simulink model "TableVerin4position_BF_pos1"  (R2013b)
settings: Solver=ode15s  StartTime=0.0  StopTime=10  RelTol=1e-3
undefined symbols (not defined in the file): deg, kg, m, mm, N, rad, s, X, Y, Z
libraries: sm_lib x907, fl_lib x24, nesl_utility x18, elec_lib x3, sdl_lib x2, simulink x1
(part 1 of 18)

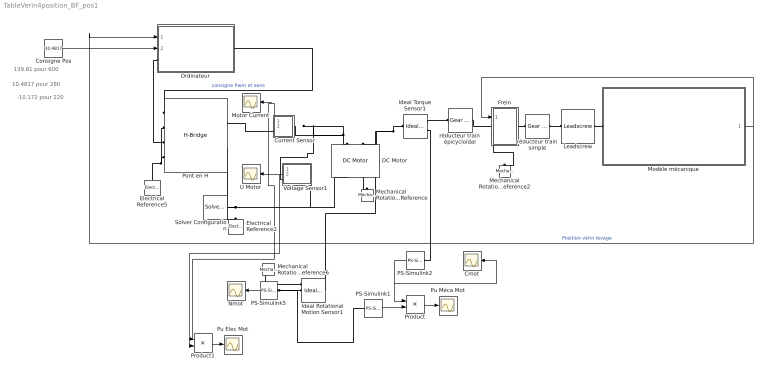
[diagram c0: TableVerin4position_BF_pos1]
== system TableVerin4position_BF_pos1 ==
  note: -10.172 pour 220
  note: 10.4817 pour 280
  note: 139.81 pour 600
  Cmot : Scope
  Consigne Pos : Constant  Value=10.4817
  Current Sensor : Subsystem
  DC Motor : elec_lib/Actuators & Drivers/Rotational Actuators/DC Motor  parameterization=1  Ra=0.53333333 Ohm  La=1600e-6 H  emf_or_torque=2  Kv=0.0637 V/rpm  Ki=0.05555555 N*m/A  T_stall=3e-3*4000/(2*pi*6.25) N*m  w_max=3250 rpm  w_rated=2375 rpm  P_rated=19 W  V_rated=24 V  J=32e-5 kg*m^2  lam_param=2  lam=1e-08 N*m/(rad/s)  i_noload=1.1 A  V_i_noload=24 V  speed0=0 rpm  current_Log=off  voltage_Log=off  power_Log=off  i2r_Log=off  torque_Log=off  speed_Log=off  LocalVarNames=|current|voltage|power|i2r|torque|speed  LocalVarDescs=|Current (A)|Voltage (V)|Power (W)|Electrical losses (W)|Torque (Nm)|Angular speed (rad/s)  LocalVarLogging=[0 0 0 0 0 0]  alpha=0.00393 1/K  Tmeas=25 C  thermal_mass=100 J/K  initial_temperature=25 C
  Electrical Reference2 : fl_lib/Electrical/Electrical Elements/Electrical Reference  i_Log=off  LocalVarNames=|i  LocalVarDescs=|i  LocalVarLogging=[]
  Electrical Reference5 : fl_lib/Electrical/Electrical Elements/Electrical Reference  i_Log=off  LocalVarNames=|i  LocalVarDescs=|i  LocalVarLogging=[]
  Frein : Subsystem
  Ideal Rotational Motion Sensor1 : fl_lib/Mechanical/Mechanical Sensors/Ideal Rotational Motion Sensor  offset=0 deg  w_Log=off  t_Log=off  phi_Log=off  LocalVarNames=|w|t|phi  LocalVarDescs=|w|t|phi  LocalVarLogging=[]
  Ideal Torque Sensor1 : fl_lib/Mechanical/Mechanical Sensors/Ideal Torque Sensor  w_Log=off  t_Log=off  LocalVarNames=|w|t  LocalVarDescs=|w|t  LocalVarLogging=[0 0]
  Leadscrew : sdl_lib/Gears/Rotational- Translational/Leadscrew  Lead=0.008 m  helix_type=1  friction_model=2  friction_parameterization=1  lambda=13 deg  alpha=14.5 deg  fr_coeff=0.08  eff_sn=0.75  eff_ns=0.45  mu_visc=0 N*m/(rad/s)  v_thr=0.001 m/s  LocalVarLogging=[]
  Mechanical Rotational Reference : fl_lib/Mechanical/Rotational Elements/Mechanical Rotational Reference  t_Log=off  LocalVarNames=|t  LocalVarDescs=|t  LocalVarLogging=[]
  Mechanical Rotational Reference2 : fl_lib/Mechanical/Rotational Elements/Mechanical Rotational Reference  t_Log=off  LocalVarNames=|t  LocalVarDescs=|t  LocalVarLogging=[]
  Mechanical Rotational Reference6 : fl_lib/Mechanical/Rotational Elements/Mechanical Rotational Reference  t_Log=off  LocalVarNames=|t  LocalVarDescs=|t  LocalVarLogging=[]
  Modèle mécanique : Subsystem
  Motor Current : Scope
  Nmot : Scope
  Ordinateur : Subsystem
  PS-Simulink1 : nesl_utility/PS-Simulink Converter  PhysicalDomain=network_engine_domain  SubClassName=ps_output  LeftPortType=input  RightPortType=output  PseudoPeriodic=off  Frequencies=[]  Unit=rad/s  AffineConversion=off
  PS-Simulink2 : nesl_utility/PS-Simulink Converter  PhysicalDomain=network_engine_domain  SubClassName=ps_output  LeftPortType=input  RightPortType=output  PseudoPeriodic=off  Frequencies=[]  Unit=N*m  AffineConversion=off
  PS-Simulink5 : nesl_utility/PS-Simulink Converter  PhysicalDomain=network_engine_domain  SubClassName=ps_output  LeftPortType=input  RightPortType=output  PseudoPeriodic=off  Frequencies=[]  Unit=rpm  AffineConversion=off
  Pont en H : elec_lib/Actuators & Drivers/Drivers/H-Bridge  Venable=2.5 V  Vmax=5 V  Vreverse=2.5 V  Vbrake=2.5 V  Vm=24 V  pwm_or_av=2  discontinuous=0  freewheeling_mode=1  freewheeling_mode_disc=1  Ron=0.1 Ohm  Don=0.1 Ohm  Rload=10 Ohm  Lload=1e-5 H  F=10 kHz  w_vec=[1, 2] s  i_vec=[1, 2] A  vMatrix=[1, 2; 3, 4] V  iENA_Log=off  iREV_Log=off  iBRK_Log=off  i2_Log=off  v_lag_Log=off  LocalVarNames=|current|voltage|power  LocalVarDescs=|Load current (A)|Load voltage (V)|Load power (W)  LocalVarLogging=[0 0 0]
  Product : Product
  Product1 : Product
  Pu Elec Mot : Scope
  Pu Méca Mot : Scope
  Solver Configuration : nesl_utility/Solver Configuration  PhysicalDomain=network_engine_domain  SubClassName=solver  LeftPortType=input  RightPortType=generic  Accelerate=off  Tones=[]  Harmonics=[]  SimulateNoise=off  Profile=off  UseLocalSampling=off  EnableSwitchedLinearOptims=on  FrequencyDomain=off  UseCCode=off  RelTol=0.001  AbsTol=1e-06  MinStep=1e-09  ToWorkspace=off  DoDC=off  ResidualTolerance=1e-09  UseLocalSolver=off  LocalSolverChoice=NE_BACKWARD_EULER_ADVANCER  LocalSolverSampleTime=0.001  DoFixedCost=off  MaxNonlinIter=3  MaxModeIter=2  LinearAlgebra=Sparse  DelaysMemoryBudget=1024
  U Motor : Scope
  Voltage Sensor1 : Subsystem
  réducteur train simple : fl_lib/Mechanical/Mechanisms/Gear Box  ratio=2.98  t_in_Log=off  t_out_Log=off  LocalVarNames=|torque_inp|ang_velocity_inp|power  LocalVarDescs=|Input shaft torque (N*m)|Input shaft angular velocity (rad/s)|Power transmitted by the box (W)  LocalVarLogging=[0 0 0]
  réducteur train épicycloïdal : fl_lib/Mechanical/Mechanisms/Gear Box  ratio=15.44  t_in_Log=off  t_out_Log=off  LocalVarNames=|torque_inp|ang_velocity_inp|power  LocalVarDescs=|Input shaft torque (N*m)|Input shaft angular velocity (rad/s)|Power transmitted by the box (W)  LocalVarLogging=[0 0 0]
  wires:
  Current Sensor/1(i) -> Product1/1, Motor Current/1
  Voltage Sensor1/2(VuMot2) -> Product1/2, U Motor/1
  Modèle mécanique/1(position) -> Frein/1(freinage), Ordinateur/1(Retour Pos)  "Position vérin levage"
  PS-Simulink2/1 -> Cmot/1, Product/1
  Product/1 -> Pu Méca Mot/1
  PS-Simulink5/1 -> Nmot/1
  PS-Simulink1/1 -> Product/2
  Product1/1 -> Pu Elec Mot/1
  Consigne Pos/1 -> Ordinateur/2(Consigne Pos)
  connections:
  DC Motor/LConn1 -- Current Sensor/LConn1 -- Voltage Sensor1/RConn1
  Leadscrew/LConn1 -- réducteur train simple/RConn1
  DC Motor/RConn2 -- Mechanical Rotational Reference/LConn1
  Frein/LConn2 -- Mechanical Rotational Reference2/LConn1
  Frein/RConn1 -- réducteur train simple/LConn1
  Leadscrew/RConn1 -- Modèle mécanique/LConn1
  Voltage Sensor1/LConn1 -- Solver Configuration/RConn1 -- Pont en H/RConn2 -- Electrical Reference2/LConn1 -- DC Motor/RConn1
  Current Sensor/RConn1 -- Pont en H/RConn1
  Pont en H/LConn2 -- Electrical Reference5/LConn1 -- Pont en H/LConn4
  Pont en H/LConn1 -- Ordinateur/RConn1  "consigne Pwm et sens"
  Ideal Torque Sensor1/LConn1 -- Ideal Rotational Motion Sensor1/LConn1 -- DC Motor/LConn2
  Ideal Torque Sensor1/RConn2 -- PS-Simulink2/LConn1
  PS-Simulink5/LConn1 -- PS-Simulink1/LConn1 -- Ideal Rotational Motion Sensor1/RConn2
  Mechanical Rotational Reference6/LConn1 -- Ideal Rotational Motion Sensor1/RConn1
  Ideal Torque Sensor1/RConn1 -- réducteur train épicycloïdal/LConn1
  réducteur train épicycloïdal/RConn1 -- Frein/LConn1
  Pont en H/LConn3 -- Ordinateur/LConn1

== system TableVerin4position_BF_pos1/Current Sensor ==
  Current Sensor : fl_lib/Electrical/Electrical Sensors/Current Sensor  i1_Log=off  v1_Log=off  LocalVarNames=|i1|v1  LocalVarDescs=|i1|v1  LocalVarLogging=[]
  PS-Simulink Converter 2 : nesl_utility/PS-Simulink Converter  PhysicalDomain=network_engine_domain  SubClassName=ps_output  LeftPortType=input  RightPortType=output  PseudoPeriodic=off  Frequencies=[]  Unit=A  AffineConversion=off
  Volts per unit current : Gain
  + : PMIOPort  Port=1  Side=Right
  - : PMIOPort  Port=2  Side=Left
  i : Outport
  V_i : Outport  Port=2
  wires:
  PS-Simulink Converter 2/1 -> Volts per unit current/1, i/1  "Current (A)"
  Volts per unit current/1 -> V_i/1  "Volts"
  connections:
  +/RConn1 -- Current Sensor/LConn1
  -/RConn1 -- Current Sensor/RConn2
  Current Sensor/RConn1 -- PS-Simulink Converter 2/LConn1

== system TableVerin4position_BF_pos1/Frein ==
  note: 240 ou 0
  freinage : Inport
  Constant1 : Constant  Value=0
  Constant2 : Constant  Value=0
  Couple1 : Scope
  Ideal Rotational Motion Sensor1 : fl_lib/Mechanical/Mechanical Sensors/Ideal Rotational Motion Sensor  offset=0 deg  w_Log=off  t_Log=off  phi_Log=off  LocalVarNames=|w|t|phi  LocalVarDescs=|w|t|phi  LocalVarLogging=[]
  Ideal Torque Sensor1 : fl_lib/Mechanical/Mechanical Sensors/Ideal Torque Sensor  w_Log=off  t_Log=off  LocalVarNames=|w|t  LocalVarDescs=|w|t  LocalVarLogging=[0 0]
  Loaded-Contact Rotational Friction : sdl_lib/Brakes & Detents/Rotational/Loaded-Contact Rotational Friction  geometry_model=1  r_eff=50 mm  d_o=150 mm  d_i=100 mm  friction_model=1  mu_coulomb=0.2  mu_w_vector=[ 0 0.1 0.2 0.3 0.4 0.5 1 2 5 10 100 1000 ] rad/s  mu_coulomb_vector=[ 0.29 0.28 0.26 0.22 0.21 0.2 0.2 0.19 0.19 0.19 0.19 0.19 ]  mu_interp_method=1  mu_extrap_method=1  mu_static=0.21  w_tol=0.001 rad/s  force_min=0.01 N  mu_visc=0 N*m/(rad/s)  initial_state_locked=0  LocalVarLogging=[]
  Mechanical Rotational Reference6 : fl_lib/Mechanical/Rotational Elements/Mechanical Rotational Reference  t_Log=off  LocalVarNames=|t  LocalVarDescs=|t  LocalVarLogging=[]
  N1 : Scope
  PS-Simulink4 : nesl_utility/PS-Simulink Converter  PhysicalDomain=network_engine_domain  SubClassName=ps_output  LeftPortType=input  RightPortType=output  PseudoPeriodic=off  Frequencies=[]  Unit=N*m  AffineConversion=off
  PS-Simulink5 : nesl_utility/PS-Simulink Converter  PhysicalDomain=network_engine_domain  SubClassName=ps_output  LeftPortType=input  RightPortType=output  PseudoPeriodic=off  Frequencies=[]  Unit=rpm  AffineConversion=off
  Simulink-PS Converter : nesl_utility/Simulink-PS Converter  PhysicalDomain=network_engine_domain  SubClassName=ps_input  LeftPortType=input  RightPortType=output  PseudoPeriodic=off  Frequencies=[]  NoiseDistribution=none  NoiseParameters=[]  Unit=N  AffineConversion=off  InputFiltering=off  SimscapeFilterOrder=1  InputFilterTimeConstant=0.001  UdotUserProvided=1
  Switch1 : Switch  Criteria=u2 > Threshold  Threshold=10.4817
  force : Scope
  out : PMIOPort  Port=1  Side=Right
  In : PMIOPort  Port=2  Side=Left
  bâti : PMIOPort  Port=3  Side=Left
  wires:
  Switch1/1 -> force/1, Simulink-PS Converter/1
  PS-Simulink5/1 -> N1/1
  PS-Simulink4/1 -> Couple1/1
  Constant1/1 -> Switch1/1
  Constant2/1 -> Switch1/3
  freinage/1 -> Switch1/2
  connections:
  PS-Simulink5/LConn1 -- Ideal Rotational Motion Sensor1/RConn2
  Ideal Torque Sensor1/RConn2 -- PS-Simulink4/LConn1
  Loaded-Contact Rotational Friction/LConn1 -- Simulink-PS Converter/RConn1
  Mechanical Rotational Reference6/LConn1 -- Ideal Rotational Motion Sensor1/RConn1
  Ideal Rotational Motion Sensor1/LConn1 -- Ideal Torque Sensor1/LConn1 -- In/RConn1
  bâti/RConn1 -- Loaded-Contact Rotational Friction/LConn2
  Loaded-Contact Rotational Friction/RConn1 -- Ideal Torque Sensor1/RConn1 -- out/RConn1

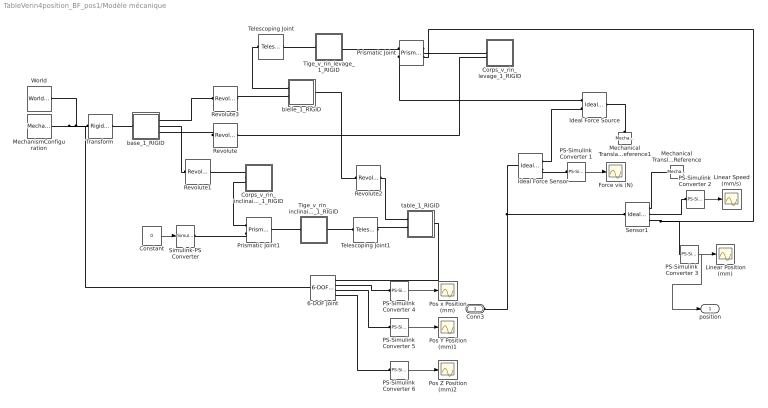
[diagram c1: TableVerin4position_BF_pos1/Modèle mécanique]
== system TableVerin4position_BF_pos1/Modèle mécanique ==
  6-DOF Joint : sm_lib/Joints/6-DOF Joint  SenseConstraintForceX=off  SenseConstraintForceY=off  SenseConstraintForceZ=off  SenseConstraintTorqueX=off  SenseConstraintTorqueY=off  SenseConstraintTorqueZ=off  ConstraintWrenchDir=FollowerOnBase  ConstraintWrenchFrame=BaseFrame  PxEquilibriumPosition=0  PxEquilibriumPositionUnits=m  PxSpringStiffness=0  PxSpringStiffnessUnits=N/m  PxDampingCoefficient=0  PxDampingCoefficientUnits=N/(m/s)  PxTorqueActuationMode=NoTorque  PxMotionActuationMode=ComputedMotion  PxSensePosition=on  PxSenseVelocity=off  PxSenseAcceleration=off  PxSenseTorqueForce=off  PxPositionTargetValue=0  PxPositionTargetValueUnits=m  PxPositionTargetSpecify=off  PxPositionTargetPriority=High  PxVelocityTargetValue=0  PxVelocityTargetValueUnits=m/s  PxVelocityTargetSpecify=off  PxVelocityTargetPriority=High  PyEquilibriumPosition=0  PyEquilibriumPositionUnits=m  PySpringStiffness=0  PySpringStiffnessUnits=N/m  PyDampingCoefficient=0  PyDampingCoefficientUnits=N/(m/s)  PyTorqueActuationMode=NoTorque  PyMotionActuationMode=ComputedMotion  PySensePosition=on  PySenseVelocity=off  PySenseAcceleration=off  PySenseTorqueForce=off  PyPositionTargetValue=0  PyPositionTargetValueUnits=m  PyPositionTargetSpecify=off  PyPositionTargetPriority=High  PyVelocityTargetValue=0  PyVelocityTargetValueUnits=m/s  PyVelocityTargetSpecify=off  PyVelocityTargetPriority=High  PzEquilibriumPosition=0  PzEquilibriumPositionUnits=m  PzSpringStiffness=0  PzSpringStiffnessUnits=N/m  PzDampingCoefficient=0  PzDampingCoefficientUnits=N/(m/s)  PzTorqueActuationMode=NoTorque  PzMotionActuationMode=ComputedMotion  PzSensePosition=on  PzSenseVelocity=off  PzSenseAcceleration=off  PzSenseTorqueForce=off  PzPositionTargetValue=0  PzPositionTargetValueUnits=m  PzPositionTargetSpecify=off  PzPositionTargetPriority=High  PzVelocityTargetValue=0  PzVelocityTargetValueUnits=m/s  PzVelocityTargetSpecify=off  PzVelocityTargetPriority=High  SphDefPosRotationMethod=None  SphDefPosRotationAngleUnits=deg  SphDefPosRotationStandardAxis=+Z  SphDefPosRotationAngle=0  SphDefPosRotationArbitraryAxis=[0 0 1]  SphDefPosFollAlignAxisA=+X  SphDefPosBaseAlignAxisA=+Y  SphDefPosFollAlignAxisB=+Y  SphDefPosBaseAlignAxisB=+Z  SphEqPosRotationMethod=None  SphEqPosRotationAngleUnits=deg  SphEqPosRotationStandardAxis=+Z  SphEqPosRotationAngle=0  SphEqPosRotationArbitraryAxis=[0 0 1]  SphEqPosFollAlignAxisA=+X  SphEqPosBaseAlignAxisA=+Y  SphEqPosFollAlignAxisB=+Y  SphEqPosBaseAlignAxisB=+Z  SphSpringStiffness=0  SphSpringStiffnessUnits=N*m/deg  SphDampingCoefficient=0  SphDampingCoefficientUnits=N*m/(deg/s)  SphActuateTorqueX=off  SphActuateTorqueY=off  SphActuateTorqueZ=off  SphActuateTorque=off  SphTorqueActuationMode=NoTorque  SphMotionActuationMode=ComputedMotion  SphActuationFrame=BaseFrame  SphSensePosition=off  SphSenseVelocityX=off  SphSenseVelocityY=off  SphSenseVelocityZ=off  SphSenseVelocity=off  SphSenseAccelerationX=off  SphSenseAccelerationY=off  SphSenseAccelerationZ=off  SphSenseAcceleration=off  SphSenseTorqueX=off  SphSenseTorqueY=off  SphSenseTorqueZ=off  SphSenseTorqueForce=off  SphSensingFrame=BaseFrame  SphPositionTargetRotationMethod=None  SphPositionTargetRotationAngleUnits=deg  SphPositionTargetRotationStandardAxis=+Z  SphPositionTargetRotationAngle=0  SphPositionTargetRotationArbitraryAxis=[0 0 1]  SphPositionTargetFollAlignAxisA=+X  SphPositionTargetBaseAlignAxisA=+Y  SphPositionTargetFollAlignAxisB=+Y  SphPositionTargetBaseAlignAxisB=+Z  SphPositionTargetSpecify=off  SphPositionTargetPriority=High  SphVelocityTargetValue=[0 0 0]  SphVelocityTargetValueUnits=deg/s  SphVelocityTargetSpecify=off  SphVelocityTargetPriority=High  SphVelocityTargetInFollowerFrame=on  BlockFunction=simmechanics.library.joints.sixdof_joint
  Constant : Constant  Value=0
  Corps_v_rin_inclinaison_1_RIGID : Subsystem
  Corps_v_rin_levage_1_RIGID : Subsystem
  Force vis (N) : Scope
  Ideal Force Sensor : fl_lib/Mechanical/Mechanical Sensors/Ideal Force Sensor  v_Log=off  f_Log=off  LocalVarNames=|v|f  LocalVarDescs=|v|f  LocalVarLogging=[0 0]
  Ideal Force Source : fl_lib/Mechanical/Mechanical Sources/Ideal Force Source  v_Log=off  f_Log=off  LocalVarNames=|v|f  LocalVarDescs=|v|f  LocalVarLogging=[0 0]
  Linear Position (mm) : Scope
  Linear Speed (mm/s) : Scope
  Mechanical Translational Reference : fl_lib/Mechanical/Translational Elements/Mechanical Translational Reference  f_Log=off  LocalVarNames=|f  LocalVarDescs=|f  LocalVarLogging=[]
  Mechanical Translational Reference1 : fl_lib/Mechanical/Translational Elements/Mechanical Translational Reference  f_Log=off  LocalVarNames=|f  LocalVarDescs=|f  LocalVarLogging=[]
  MechanismConfiguration : sm_lib/Utilities/Mechanism Configuration  GravityVector=[0 0 -9.81]  GravityUnits=m/s^2  AllowGravitySignal=off  LinearizationDelta=0.001  BlockFunction=simmechanics.library.utilities.mechanism_configuration
  PS-Simulink Converter 1 : nesl_utility/PS-Simulink Converter  PhysicalDomain=network_engine_domain  SubClassName=ps_output  LeftPortType=input  RightPortType=output  PseudoPeriodic=off  Frequencies=[]  Unit=N  AffineConversion=off
  PS-Simulink Converter 2 : nesl_utility/PS-Simulink Converter  PhysicalDomain=network_engine_domain  SubClassName=ps_output  LeftPortType=input  RightPortType=output  PseudoPeriodic=off  Frequencies=[]  Unit=mm/s  AffineConversion=off
  PS-Simulink Converter {3..6} (4 alike) : nesl_utility/PS-Simulink Converter  PhysicalDomain=network_engine_domain  SubClassName=ps_output  LeftPortType=input  RightPortType=output  PseudoPeriodic=off  Frequencies=[]  Unit=mm  AffineConversion=off
  Pos Y Position (mm)1 : Scope
  Pos Z Position (mm)2 : Scope
  Pos x Position (mm) : Scope
  Prismatic Joint : sm_lib/Joints/Prismatic Joint  SenseConstraintForceX=off  SenseConstraintForceY=off  SenseConstraintForceZ=off  SenseConstraintTorqueX=off  SenseConstraintTorqueY=off  SenseConstraintTorqueZ=off  ConstraintWrenchDir=FollowerOnBase  ConstraintWrenchFrame=BaseFrame  EquilibriumPosition=0  EquilibriumPositionUnits=m  SpringStiffness=0  SpringStiffnessUnits=N/m  DampingCoefficient=0  DampingCoefficientUnits=N/(m/s)  TorqueActuationMode=ComputedTorque  MotionActuationMode=InputMotion  SensePosition=off  SenseVelocity=off  SenseAcceleration=off  SenseTorqueForce=on  PositionTargetValue=0  PositionTargetValueUnits=m  PositionTargetSpecify=off  PositionTargetPriority=High  VelocityTargetValue=0  VelocityTargetValueUnits=m/s  VelocityTargetSpecify=off  VelocityTargetPriority=High  BlockFunction=simmechanics.library.joints.prismatic_joint
  Prismatic Joint1 : sm_lib/Joints/Prismatic Joint  SenseConstraintForceX=off  SenseConstraintForceY=off  SenseConstraintForceZ=off  SenseConstraintTorqueX=off  SenseConstraintTorqueY=off  SenseConstraintTorqueZ=off  ConstraintWrenchDir=FollowerOnBase  ConstraintWrenchFrame=BaseFrame  EquilibriumPosition=0  EquilibriumPositionUnits=m  SpringStiffness=0  SpringStiffnessUnits=N/m  DampingCoefficient=0  DampingCoefficientUnits=N/(m/s)  TorqueActuationMode=ComputedTorque  MotionActuationMode=InputMotion  SensePosition=off  SenseVelocity=off  SenseAcceleration=off  SenseTorqueForce=off  PositionTargetValue=0  PositionTargetValueUnits=m  PositionTargetSpecify=off  PositionTargetPriority=High  VelocityTargetValue=0  VelocityTargetValueUnits=m/s  VelocityTargetSpecify=off  VelocityTargetPriority=High  BlockFunction=simmechanics.library.joints.prismatic_joint
  Revolute : sm_lib/Joints/Revolute Joint  SenseConstraintForceX=off  SenseConstraintForceY=off  SenseConstraintForceZ=off  SenseConstraintTorqueX=off  SenseConstraintTorqueY=off  SenseConstraintTorqueZ=off  ConstraintWrenchDir=FollowerOnBase  ConstraintWrenchFrame=BaseFrame  EquilibriumPosition=0  EquilibriumPositionUnits=rad  SpringStiffness=0  SpringStiffnessUnits=m*N/rad  DampingCoefficient=0  DampingCoefficientUnits=m*s*N/rad  TorqueActuationMode=NoTorque  MotionActuationMode=ComputedMotion  SensePosition=off  SenseVelocity=off  SenseAcceleration=off  SenseTorqueForce=off  PositionTargetValue=-19.448954484523508  PositionTargetValueUnits=deg  PositionTargetSpecify=on  PositionTargetPriority=Low  VelocityTargetValue=0  VelocityTargetValueUnits=deg/s  VelocityTargetSpecify=off  VelocityTargetPriority=High  BlockFunction=simmechanics.library.joints.revolute_joint
  Revolute1 : sm_lib/Joints/Revolute Joint  SenseConstraintForceX=off  SenseConstraintForceY=off  SenseConstraintForceZ=off  SenseConstraintTorqueX=off  SenseConstraintTorqueY=off  SenseConstraintTorqueZ=off  ConstraintWrenchDir=FollowerOnBase  ConstraintWrenchFrame=BaseFrame  EquilibriumPosition=0  EquilibriumPositionUnits=rad  SpringStiffness=0  SpringStiffnessUnits=m*N/rad  DampingCoefficient=0  DampingCoefficientUnits=m*s*N/rad  TorqueActuationMode=NoTorque  MotionActuationMode=ComputedMotion  SensePosition=off  SenseVelocity=off  SenseAcceleration=off  SenseTorqueForce=off  PositionTargetValue=-0.69151960924487288  PositionTargetValueUnits=deg  PositionTargetSpecify=on  PositionTargetPriority=Low  VelocityTargetValue=0  VelocityTargetValueUnits=deg/s  VelocityTargetSpecify=off  VelocityTargetPriority=High  BlockFunction=simmechanics.library.joints.revolute_joint
  Revolute2 : sm_lib/Joints/Revolute Joint  SenseConstraintForceX=off  SenseConstraintForceY=off  SenseConstraintForceZ=off  SenseConstraintTorqueX=off  SenseConstraintTorqueY=off  SenseConstraintTorqueZ=off  ConstraintWrenchDir=FollowerOnBase  ConstraintWrenchFrame=BaseFrame  EquilibriumPosition=0  EquilibriumPositionUnits=rad  SpringStiffness=0  SpringStiffnessUnits=m*N/rad  DampingCoefficient=0  DampingCoefficientUnits=m*s*N/rad  TorqueActuationMode=NoTorque  MotionActuationMode=ComputedMotion  SensePosition=off  SenseVelocity=off  SenseAcceleration=off  SenseTorqueForce=off  PositionTargetValue=37.808774161373094  PositionTargetValueUnits=deg  PositionTargetSpecify=on  PositionTargetPriority=Low  VelocityTargetValue=0  VelocityTargetValueUnits=deg/s  VelocityTargetSpecify=off  VelocityTargetPriority=High  BlockFunction=simmechanics.library.joints.revolute_joint
  Revolute3 : sm_lib/Joints/Revolute Joint  SenseConstraintForceX=off  SenseConstraintForceY=off  SenseConstraintForceZ=off  SenseConstraintTorqueX=off  SenseConstraintTorqueY=off  SenseConstraintTorqueZ=off  ConstraintWrenchDir=FollowerOnBase  ConstraintWrenchFrame=BaseFrame  EquilibriumPosition=0  EquilibriumPositionUnits=rad  SpringStiffness=0  SpringStiffnessUnits=m*N/rad  DampingCoefficient=0  DampingCoefficientUnits=m*s*N/rad  TorqueActuationMode=NoTorque  MotionActuationMode=ComputedMotion  SensePosition=off  SenseVelocity=off  SenseAcceleration=off  SenseTorqueForce=off  PositionTargetValue=-37.808774161373101  PositionTargetValueUnits=deg  PositionTargetSpecify=on  PositionTargetPriority=Low  VelocityTargetValue=0  VelocityTargetValueUnits=deg/s  VelocityTargetSpecify=off  VelocityTargetPriority=High  BlockFunction=simmechanics.library.joints.revolute_joint
  Sensor1 : fl_lib/Mechanical/Mechanical Sensors/Ideal Translational Motion Sensor  offset=0 m  v_Log=off  f_Log=off  x_Log=off  LocalVarNames=|v|f|x  LocalVarDescs=|v|f|x  LocalVarLogging=[]
  Simulink-PS Converter : nesl_utility/Simulink-PS Converter  PhysicalDomain=network_engine_domain  SubClassName=ps_input  LeftPortType=input  RightPortType=output  PseudoPeriodic=off  Frequencies=[]  NoiseDistribution=none  NoiseParameters=[]  Unit=m  AffineConversion=off  InputFiltering=off  SimscapeFilterOrder=1  InputFilterTimeConstant=0.001  UdotUserProvided=1
  Telescoping Joint : sm_lib/Joints/Telescoping Joint  SenseConstraintForceX=off  SenseConstraintForceY=off  SenseConstraintForceZ=off  SenseConstraintTorqueX=off  SenseConstraintTorqueY=off  SenseConstraintTorqueZ=off  ConstraintWrenchDir=FollowerOnBase  ConstraintWrenchFrame=BaseFrame  SphDefPosRotationMethod=None  SphDefPosRotationAngleUnits=deg  SphDefPosRotationStandardAxis=+Z  SphDefPosRotationAngle=0  SphDefPosRotationArbitraryAxis=[0 0 1]  SphDefPosFollAlignAxisA=+X  SphDefPosBaseAlignAxisA=+Y  SphDefPosFollAlignAxisB=+Y  SphDefPosBaseAlignAxisB=+Z  SphEqPosRotationMethod=None  SphEqPosRotationAngleUnits=deg  SphEqPosRotationStandardAxis=+Z  SphEqPosRotationAngle=0  SphEqPosRotationArbitraryAxis=[0 0 1]  SphEqPosFollAlignAxisA=+X  SphEqPosBaseAlignAxisA=+Y  SphEqPosFollAlignAxisB=+Y  SphEqPosBaseAlignAxisB=+Z  SphSpringStiffness=0  SphSpringStiffnessUnits=N*m/deg  SphDampingCoefficient=0  SphDampingCoefficientUnits=N*m/(deg/s)  SphActuateTorqueX=off  SphActuateTorqueY=off  SphActuateTorqueZ=off  SphActuateTorque=off  SphTorqueActuationMode=NoTorque  SphMotionActuationMode=ComputedMotion  SphActuationFrame=BaseFrame  SphSensePosition=off  SphSenseVelocityX=off  SphSenseVelocityY=off  SphSenseVelocityZ=off  SphSenseVelocity=off  SphSenseAccelerationX=off  SphSenseAccelerationY=off  SphSenseAccelerationZ=off  SphSenseAcceleration=off  SphSenseTorqueX=off  SphSenseTorqueY=off  SphSenseTorqueZ=off  SphSenseTorqueForce=off  SphSensingFrame=BaseFrame  SphPositionTargetRotationMethod=None  SphPositionTargetRotationAngleUnits=deg  SphPositionTargetRotationStandardAxis=+Z  SphPositionTargetRotationAngle=0  SphPositionTargetRotationArbitraryAxis=[0 0 1]  SphPositionTargetFollAlignAxisA=+X  SphPositionTargetBaseAlignAxisA=+Y  SphPositionTargetFollAlignAxisB=+Y  SphPositionTargetBaseAlignAxisB=+Z  SphPositionTargetSpecify=off  SphPositionTargetPriority=High  SphVelocityTargetValue=[0 0 0]  SphVelocityTargetValueUnits=deg/s  SphVelocityTargetSpecify=off  SphVelocityTargetPriority=High  SphVelocityTargetInFollowerFrame=on  PzEquilibriumPosition=0  PzEquilibriumPositionUnits=m  PzSpringStiffness=0  PzSpringStiffnessUnits=N/m  PzDampingCoefficient=0  PzDampingCoefficientUnits=N/(m/s)  PzTorqueActuationMode=NoTorque  PzMotionActuationMode=ComputedMotion  PzSensePosition=off  PzSenseVelocity=off  PzSenseAcceleration=off  PzSenseTorqueForce=off  PzPositionTargetValue=0  PzPositionTargetValueUnits=m  PzPositionTargetSpecify=off  PzPositionTargetPriority=High  PzVelocityTargetValue=0  PzVelocityTargetValueUnits=m/s  PzVelocityTargetSpecify=off  PzVelocityTargetPriority=High  BlockFunction=simmechanics.library.joints.telescoping_joint
  Telescoping Joint1 : sm_lib/Joints/Telescoping Joint  SenseConstraintForceX=off  SenseConstraintForceY=off  SenseConstraintForceZ=off  SenseConstraintTorqueX=off  SenseConstraintTorqueY=off  SenseConstraintTorqueZ=off  ConstraintWrenchDir=FollowerOnBase  ConstraintWrenchFrame=BaseFrame  SphDefPosRotationMethod=None  SphDefPosRotationAngleUnits=deg  SphDefPosRotationStandardAxis=+Z  SphDefPosRotationAngle=0  SphDefPosRotationArbitraryAxis=[0 0 1]  SphDefPosFollAlignAxisA=+X  SphDefPosBaseAlignAxisA=+Y  SphDefPosFollAlignAxisB=+Y  SphDefPosBaseAlignAxisB=+Z  SphEqPosRotationMethod=None  SphEqPosRotationAngleUnits=deg  SphEqPosRotationStandardAxis=+Z  SphEqPosRotationAngle=0  SphEqPosRotationArbitraryAxis=[0 0 1]  SphEqPosFollAlignAxisA=+X  SphEqPosBaseAlignAxisA=+Y  SphEqPosFollAlignAxisB=+Y  SphEqPosBaseAlignAxisB=+Z  SphSpringStiffness=0  SphSpringStiffnessUnits=N*m/deg  SphDampingCoefficient=0  SphDampingCoefficientUnits=N*m/(deg/s)  SphActuateTorqueX=off  SphActuateTorqueY=off  SphActuateTorqueZ=off  SphActuateTorque=off  SphTorqueActuationMode=NoTorque  SphMotionActuationMode=ComputedMotion  SphActuationFrame=BaseFrame  SphSensePosition=off  SphSenseVelocityX=off  SphSenseVelocityY=off  SphSenseVelocityZ=off  SphSenseVelocity=off  SphSenseAccelerationX=off  SphSenseAccelerationY=off  SphSenseAccelerationZ=off  SphSenseAcceleration=off  SphSenseTorqueX=off  SphSenseTorqueY=off  SphSenseTorqueZ=off  SphSenseTorqueForce=off  SphSensingFrame=BaseFrame  SphPositionTargetRotationMethod=None  SphPositionTargetRotationAngleUnits=deg  SphPositionTargetRotationStandardAxis=+Z  SphPositionTargetRotationAngle=0  SphPositionTargetRotationArbitraryAxis=[0 0 1]  SphPositionTargetFollAlignAxisA=+X  SphPositionTargetBaseAlignAxisA=+Y  SphPositionTargetFollAlignAxisB=+Y  SphPositionTargetBaseAlignAxisB=+Z  SphPositionTargetSpecify=off  SphPositionTargetPriority=High  SphVelocityTargetValue=[0 0 0]  SphVelocityTargetValueUnits=deg/s  SphVelocityTargetSpecify=off  SphVelocityTargetPriority=High  SphVelocityTargetInFollowerFrame=on  PzEquilibriumPosition=0  PzEquilibriumPositionUnits=m  PzSpringStiffness=0  PzSpringStiffnessUnits=N/m  PzDampingCoefficient=0  PzDampingCoefficientUnits=N/(m/s)  PzTorqueActuationMode=NoTorque  PzMotionActuationMode=ComputedMotion  PzSensePosition=off  PzSenseVelocity=off  PzSenseAcceleration=off  PzSenseTorqueForce=off  PzPositionTargetValue=0  PzPositionTargetValueUnits=m  PzPositionTargetSpecify=off  PzPositionTargetPriority=High  PzVelocityTargetValue=0  PzVelocityTargetValueUnits=m/s  PzVelocityTargetSpecify=off  PzVelocityTargetPriority=High  BlockFunction=simmechanics.library.joints.telescoping_joint
  Tige_v_rin_inclinaison_1_RIGID : Subsystem
  Tige_v_rin_levage_1_RIGID : Subsystem
  Transform : sm_lib/Frames and Transforms/Rigid Transform  TranslationMethod=Cartesian  TranslationLengthUnit=mm  TranslationStandardAxis=+Z  TranslationStandardOffset=0  TranslationCartesianOffset=[-44.940899999999999 -2.2279000000000001e-11 85]  TranslationROffset=0  TranslationROffsetUnits=m  TranslationZOffset=0  TranslationZOffsetUnits=m  TranslationThetaOffset=0  TranslationThetaOffsetUnits=deg  RotationMethod=None  RotationAngleUnits=deg  RotationStandardAxis=+Z  RotationAngle=0  RotationArbitraryAxis=[0 0 1]  FollAlignAxisA=+X  BaseAlignAxisA=+Y  FollAlignAxisB=+Y  BaseAlignAxisB=+Z  BlockFunction=simmechanics.library.frames_transforms.rigid_transform
  World : sm_lib/Frames and Transforms/World Frame  BlockFunction=simmechanics.library.frames_transforms.world_frame
  base_1_RIGID : Subsystem
  bielle_1_RIGID : Subsystem
  table_1_RIGID : Subsystem
  Conn3 : PMIOPort  Port=1  Side=Left
  position : Outport
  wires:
  Constant/1 -> Simulink-PS Converter/1
  PS-Simulink Converter 3/1 -> position/1, Linear Position (mm)/1
  PS-Simulink Converter 2/1 -> Linear Speed (mm/s)/1
  PS-Simulink Converter 1/1 -> Force vis (N)/1
  PS-Simulink Converter 4/1 -> Pos x Position (mm)/1
  PS-Simulink Converter 5/1 -> Pos Y Position (mm)1/1
  PS-Simulink Converter 6/1 -> Pos Z Position (mm)2/1
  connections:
  Revolute/LConn1 -- base_1_RIGID/RConn3
  MechanismConfiguration/RConn1 -- World/RConn1 -- 6-DOF Joint/LConn1 -- Transform/LConn1
  Revolute2/RConn1 -- table_1_RIGID/LConn1
  Revolute2/LConn1 -- bielle_1_RIGID/RConn1
  Corps_v_rin_levage_1_RIGID/LConn2 -- Revolute/RConn1
  Prismatic Joint1/RConn1 -- Tige_v_rin_inclinaison_1_RIGID/RConn1
  Transform/RConn1 -- base_1_RIGID/LConn1
  Revolute3/RConn1 -- bielle_1_RIGID/LConn2
  Revolute3/LConn1 -- base_1_RIGID/RConn1
  Prismatic Joint1/LConn1 -- Corps_v_rin_inclinaison_1_RIGID/LConn2
  bielle_1_RIGID/LConn1 -- Telescoping Joint/LConn1
  Telescoping Joint/RConn1 -- Tige_v_rin_levage_1_RIGID/LConn1
  Sensor1/LConn1 -- Ideal Force Sensor/LConn1 -- Conn3/RConn1
  Telescoping Joint1/RConn1 -- table_1_RIGID/LConn2
  Tige_v_rin_inclinaison_1_RIGID/LConn1 -- Telescoping Joint1/LConn1
  Ideal Force Source/RConn1 -- Prismatic Joint/RConn2
  Prismatic Joint/LConn1 -- Corps_v_rin_levage_1_RIGID/LConn1
  Corps_v_rin_inclinaison_1_RIGID/LConn1 -- Revolute1/RConn1
  Mechanical Translational Reference1/LConn1 -- Ideal Force Source/LConn1
  Tige_v_rin_levage_1_RIGID/RConn1 -- Prismatic Joint/RConn1
  Revolute1/LConn1 -- base_1_RIGID/RConn2
  Prismatic Joint1/LConn2 -- Simulink-PS Converter/RConn1
  Prismatic Joint/LConn2 -- PS-Simulink Converter 3/LConn1 -- Sensor1/RConn3
  Sensor1/RConn1 -- Mechanical Translational Reference/LConn1
  PS-Simulink Converter 2/LConn1 -- Sensor1/RConn2
  Ideal Force Sensor/RConn2 -- PS-Simulink Converter 1/LConn1
  Ideal Force Sensor/RConn1 -- Ideal Force Source/RConn2
  6-DOF Joint/RConn1 -- table_1_RIGID/RConn1
  6-DOF Joint/RConn2 -- PS-Simulink Converter 4/LConn1
  PS-Simulink Converter 5/LConn1 -- 6-DOF Joint/RConn3
  PS-Simulink Converter 6/LConn1 -- 6-DOF Joint/RConn4

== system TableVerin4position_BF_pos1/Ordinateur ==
  Retour Pos : Inport
  Consigne Pos : Inport  Port=2
  5/140 : Gain  Gain=5/140
  5/140. : Gain  Gain=5/140
  Abs : Abs
  ConsVitesse1 : Scope
  Constant1 : Constant  Value=0
  Constant2 : Constant  Value=5
  Controlled PWM Voltage : elec_lib/Actuators & Drivers/Drivers/Controlled PWM Voltage  F=10000 Hz  TD=0 s  pulse_width_offset=0 s  Vmin=0 V  Vmax=5 V  Vm=5 V  pwm_or_av=2  event_type=1  sample_time=1e-6 s  LocalVarNames=|current|voltage|power  LocalVarDescs=|Load current (A)|Load voltage (V)|Load power (W)  LocalVarLogging=[0 0 0]
  Controlled Voltage Source : fl_lib/Electrical/Electrical Sources/Controlled Voltage Source  i_Log=off  v_Log=off  LocalVarNames=|i|v  LocalVarDescs=|i|v  LocalVarLogging=[0 0]
  Controlled Voltage Source1 : fl_lib/Electrical/Electrical Sources/Controlled Voltage Source  i_Log=off  v_Log=off  LocalVarNames=|i|v  LocalVarDescs=|i|v  LocalVarLogging=[0 0]
  Electrical Reference1 : fl_lib/Electrical/Electrical Elements/Electrical Reference  i_Log=off  LocalVarNames=|i  LocalVarDescs=|i  LocalVarLogging=[]
  Electrical Reference3 : fl_lib/Electrical/Electrical Elements/Electrical Reference  i_Log=off  LocalVarNames=|i  LocalVarDescs=|i  LocalVarLogging=[]
  Electrical Reference4 : fl_lib/Electrical/Electrical Elements/Electrical Reference  i_Log=off  LocalVarNames=|i  LocalVarDescs=|i  LocalVarLogging=[]
  PID : Scope
  PID Controller : simulink/Continuous/PID Controller  Controller=PID  TimeDomain=Continuous-time  SampleTime=1  IntegratorMethod=Forward Euler  FilterMethod=Forward Euler  Form=Parallel  P=50  I=20  D=75  N=100  InitialConditionSource=internal  InitialConditionForIntegrator=0  InitialConditionForFilter=0  ExternalReset=none  LimitOutput=off  UpperSaturationLimit=inf  LowerSaturationLimit=-inf  LinearizeAsGain=on  AntiWindupMode=none  Kb=1  TrackingMode=off  Kt=1  PParamMin=[]  PParamMax=[]  IParamMin=[]  IParamMax=[]  DParamMin=[]  DParamMax=[]  NParamMin=[]  NParamMax=[]  KbParamMin=[]  KbParamMax=[]  KtParamMin=[]  KtParamMax=[]  POutMin=[]  POutMax=[]  IOutMin=[]  IOutMax=[]  DOutMin=[]  DOutMax=[]  NOutMin=[]  NOutMax=[]  KbOutMin=[]  KbOutMax=[]  KtOutMin=[]  KtOutMax=[]  IntegratorOutMin=[]  IntegratorOutMax=[]  FilterOutMin=[]  FilterOutMax=[]  SumOutMin=[]  SumOutMax=[]  SumI1OutMin=[]  SumI1OutMax=[]  SumI2OutMin=[]  SumI2OutMax=[]  SumI3OutMin=[]  SumI3OutMax=[]  SumDOutMin=[]  SumDOutMax=[]  SaturationOutMin=[]  SaturationOutMax=[]  IntegratorContinuousStateAttributes=''  IntegratorStateMustResolveToSignalObject=off  IntegratorRTWStateStorageClass=Auto  FilterContinuousStateAttributes=''  FilterStateMustResolveToSignalObject=off  FilterRTWStateStorageClass=Auto
  Saturation vitesse : Saturate  UpperLimit=5  LowerLimit=0
  Sens Vitesse : Scope
  Simulink-PS Converter : nesl_utility/Simulink-PS Converter  PhysicalDomain=network_engine_domain  SubClassName=ps_input  LeftPortType=input  RightPortType=output  PseudoPeriodic=off  Frequencies=[]  NoiseDistribution=none  NoiseParameters=[]  Unit=V  AffineConversion=off  InputFiltering=off  SimscapeFilterOrder=1  InputFilterTimeConstant=0.001  UdotUserProvided=1
  Simulink-PS Converter1 : nesl_utility/Simulink-PS Converter  PhysicalDomain=network_engine_domain  SubClassName=ps_input  LeftPortType=input  RightPortType=output  PseudoPeriodic=off  Frequencies=[]  NoiseDistribution=none  NoiseParameters=[]  Unit=V  AffineConversion=off  InputFiltering=off  SimscapeFilterOrder=1  InputFilterTimeConstant=0.001  UdotUserProvided=1
  Sum : Sum  Inputs=|+-
  Switch : Switch
  erreur : Scope
  Tension : PMIOPort  Port=1  Side=Right
  Sens : PMIOPort  Port=2  Side=Left
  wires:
  Saturation vitesse/1 -> Simulink-PS Converter/1, ConsVitesse1/1
  PID Controller/1 -> PID/1, Switch/2, Abs/1
  Sum/1 -> PID Controller/1, erreur/1
  Switch/1 -> Sens Vitesse/1, Simulink-PS Converter1/1
  Consigne Pos/1 -> 5/140./1
  5/140./1 -> Sum/1
  Retour Pos/1 -> 5/140/1
  5/140/1 -> Sum/2
  Abs/1 -> Saturation vitesse/1
  Constant1/1 -> Switch/1
  Constant2/1 -> Switch/3
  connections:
  Controlled Voltage Source/LConn1 -- Controlled PWM Voltage/LConn1
  Tension/RConn1 -- Controlled PWM Voltage/RConn1
  Controlled PWM Voltage/RConn2 -- Controlled PWM Voltage/LConn2 -- Electrical Reference1/LConn1
  Simulink-PS Converter/RConn1 -- Controlled Voltage Source/RConn1
  Electrical Reference3/LConn1 -- Controlled Voltage Source/RConn2
  Electrical Reference4/LConn1 -- Controlled Voltage Source1/RConn2
  Controlled Voltage Source1/LConn1 -- Sens/RConn1
  Simulink-PS Converter1/RConn1 -- Controlled Voltage Source1/RConn1

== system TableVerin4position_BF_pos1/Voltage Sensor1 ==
  PS-Simulink Converter 2 : nesl_utility/PS-Simulink Converter  PhysicalDomain=network_engine_domain  SubClassName=ps_output  LeftPortType=input  RightPortType=output  PseudoPeriodic=off  Frequencies=[]  Unit=V  AffineConversion=off
  Voltage Sensor : fl_lib/Electrical/Electrical Sensors/Voltage Sensor  i1_Log=off  v1_Log=off  LocalVarNames=|i1|v1  LocalVarDescs=|i1|v1  LocalVarLogging=[0 0]
  + : PMIOPort  Port=1  Side=Right
  - : PMIOPort  Port=2  Side=Left
  uMot : Outport
  VuMot2 : Outport  Port=2
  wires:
  PS-Simulink Converter 2/1 -> VuMot2/1, uMot/1  "Tension (V)"
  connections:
  Voltage Sensor/LConn1 -- +/RConn1
  -/RConn1 -- Voltage Sensor/RConn2
  Voltage Sensor/RConn1 -- PS-Simulink Converter 2/LConn1

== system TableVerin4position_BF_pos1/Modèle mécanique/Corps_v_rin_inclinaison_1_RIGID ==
  ReferenceFrame : sm_lib/Frames and Transforms/Reference Frame  BlockFunction=simmechanics.library.frames_transforms.reference_frame
  Transform : sm_lib/Frames and Transforms/Rigid Transform  TranslationMethod=Cartesian  TranslationLengthUnit=mm  TranslationStandardAxis=+Z  TranslationStandardOffset=0  TranslationCartesianOffset=[581.58897838011512 -79.972299999999905 18.779086684198781]  TranslationROffset=0  TranslationROffsetUnits=m  TranslationZOffset=0  TranslationZOffsetUnits=m  TranslationThetaOffset=0  TranslationThetaOffsetUnits=deg  RotationMethod=ArbitraryAxis  RotationAngleUnits=rad  RotationStandardAxis=+Z  RotationAngle=2.0943951023931957  RotationArbitraryAxis=[0.57735026918962573 0.57735026918962584 0.57735026918962573]  FollAlignAxisA=+X  BaseAlignAxisA=+Y  FollAlignAxisB=+Y  BaseAlignAxisB=+Z  BlockFunction=simmechanics.library.frames_transforms.rigid_transform
  Transform1 : sm_lib/Frames and Transforms/Rigid Transform  TranslationMethod=Cartesian  TranslationLengthUnit=mm  TranslationStandardAxis=+Z  TranslationStandardOffset=0  TranslationCartesianOffset=[16.943688345754151 -124.27970000002227 18.779161135203918]  TranslationROffset=0  TranslationROffsetUnits=m  TranslationZOffset=0  TranslationZOffsetUnits=m  TranslationThetaOffset=0  TranslationThetaOffsetUnits=deg  RotationMethod=ArbitraryAxis  RotationAngleUnits=rad  RotationStandardAxis=+Z  RotationAngle=2.0943951023931957  RotationArbitraryAxis=[0.57735026918962584 -0.57735026918962551 0.57735026918962595]  FollAlignAxisA=+X  BaseAlignAxisA=+Y  FollAlignAxisB=+Y  BaseAlignAxisB=+Z  BlockFunction=simmechanics.library.frames_transforms.rigid_transform
  Transform2 : sm_lib/Frames and Transforms/Rigid Transform  TranslationMethod=Cartesian  TranslationLengthUnit=mm  TranslationStandardAxis=+Z  TranslationStandardOffset=0  TranslationCartesianOffset=[223.357 -79.97229999999999 92.199100000000001]  TranslationROffset=0  TranslationROffsetUnits=m  TranslationZOffset=0  TranslationZOffsetUnits=m  TranslationThetaOffset=0  TranslationThetaOffsetUnits=deg  RotationMethod=ArbitraryAxis  RotationAngleUnits=rad  RotationStandardAxis=+Z  RotationAngle=3.1415926535897931  RotationArbitraryAxis=[-0.70710678118654746 -5.2401915786782071e-17 -0.70710678118654757]  FollAlignAxisA=+X  BaseAlignAxisA=+Y  FollAlignAxisB=+Y  BaseAlignAxisB=+Z  BlockFunction=simmechanics.library.frames_transforms.rigid_transform
  Transform3 : sm_lib/Frames and Transforms/Rigid Transform  TranslationMethod=Cartesian  TranslationLengthUnit=mm  TranslationStandardAxis=+Z  TranslationStandardOffset=0  TranslationCartesianOffset=[61.256599999999999 -79.97229999999999 18.7791]  TranslationROffset=0  TranslationROffsetUnits=m  TranslationZOffset=0  TranslationZOffsetUnits=m  TranslationThetaOffset=0  TranslationThetaOffsetUnits=deg  RotationMethod=ArbitraryAxis  RotationAngleUnits=rad  RotationStandardAxis=+Z  RotationAngle=1.6178481128137681  RotationArbitraryAxis=[0.21194708467810194 -0.21194708467810194 0.95402141830930975]  FollAlignAxisA=+X  BaseAlignAxisA=+Y  FollAlignAxisB=+Y  BaseAlignAxisB=+Z  BlockFunction=simmechanics.library.frames_transforms.rigid_transform
  Transform4 : sm_lib/Frames and Transforms/Rigid Transform  TranslationMethod=Cartesian  TranslationLengthUnit=mm  TranslationStandardAxis=+Z  TranslationStandardOffset=0  TranslationCartesianOffset=[16.944099999999999 -79.97229999999999 18.7791]  TranslationROffset=0  TranslationROffsetUnits=m  TranslationZOffset=0  TranslationZOffsetUnits=m  TranslationThetaOffset=0  TranslationThetaOffsetUnits=deg  RotationMethod=None  RotationAngleUnits=deg  RotationStandardAxis=+Z  RotationAngle=0  RotationArbitraryAxis=[0 0 1]  FollAlignAxisA=+X  BaseAlignAxisA=+Y  FollAlignAxisB=+Y  BaseAlignAxisB=+Z  BlockFunction=simmechanics.library.frames_transforms.rigid_transform
  Transform5 : sm_lib/Frames and Transforms/Rigid Transform  TranslationMethod=Cartesian  TranslationLengthUnit=mm  TranslationStandardAxis=+Z  TranslationStandardOffset=0  TranslationCartesianOffset=[117.25700000000001 -79.97229999999999 18.7791]  TranslationROffset=0  TranslationROffsetUnits=m  TranslationZOffset=0  TranslationZOffsetUnits=m  TranslationThetaOffset=0  TranslationThetaOffsetUnits=deg  RotationMethod=ArbitraryAxis  RotationAngleUnits=rad  RotationStandardAxis=+Z  RotationAngle=3.1415926535897931  RotationArbitraryAxis=[0 0.97311979050629582 0.2302995295804641]  FollAlignAxisA=+X  BaseAlignAxisA=+Y  FollAlignAxisB=+Y  BaseAlignAxisB=+Z  BlockFunction=simmechanics.library.frames_transforms.rigid_transform
  x15060_Ecrou_24_Ecrou_Hm_M16_1_RIGID : Subsystem
  x15060_M_01073_Interface_ar_verin_AA_DEFAULT_1_RIGID : Subsystem
  x15060_NLM_Embout_a_rotule_M16_Pas_a_droite_27627_16_1_RIGID : Subsystem
  x15060_Verin_LA36_Course_100_mm_1_RIGID : Subsystem
  F1 : PMIOPort  Port=1  Side=Left
  F : PMIOPort  Port=2  Side=Left
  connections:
  Transform/LConn1 -- ReferenceFrame/RConn1 -- Transform1/LConn1 -- Transform2/LConn1 -- Transform3/LConn1 -- Transform4/LConn1 -- Transform5/LConn1
  Transform/RConn1 -- F/RConn1
  Transform1/RConn1 -- F1/RConn1
  Transform2/RConn1 -- x15060_Verin_LA36_Course_100_mm_1_RIGID/LConn1
  Transform3/RConn1 -- x15060_Ecrou_24_Ecrou_Hm_M16_1_RIGID/LConn1
  Transform4/RConn1 -- x15060_NLM_Embout_a_rotule_M16_Pas_a_droite_27627_16_1_RIGID/LConn1
  Transform5/RConn1 -- x15060_M_01073_Interface_ar_verin_AA_DEFAULT_1_RIGID/LConn1

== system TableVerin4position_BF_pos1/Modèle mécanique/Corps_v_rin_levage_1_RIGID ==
  ReferenceFrame : sm_lib/Frames and Transforms/Reference Frame  BlockFunction=simmechanics.library.frames_transforms.reference_frame
  Transform : sm_lib/Frames and Transforms/Rigid Transform  TranslationMethod=Cartesian  TranslationLengthUnit=mm  TranslationStandardAxis=+Z  TranslationStandardOffset=0  TranslationCartesianOffset=[16.948520761169686 32.492699999977624 18.777580013894262]  TranslationROffset=0  TranslationROffsetUnits=m  TranslationZOffset=0  TranslationZOffsetUnits=m  TranslationThetaOffset=0  TranslationThetaOffsetUnits=deg  RotationMethod=ArbitraryAxis  RotationAngleUnits=rad  RotationStandardAxis=+Z  RotationAngle=2.0943951023931935  RotationArbitraryAxis=[-0.57735026918962506 -0.57735026918962595 -0.5773502691896264]  FollAlignAxisA=+X  BaseAlignAxisA=+Y  FollAlignAxisB=+Y  BaseAlignAxisB=+Z  BlockFunction=simmechanics.library.frames_transforms.rigid_transform
  Transform1 : sm_lib/Frames and Transforms/Rigid Transform  TranslationMethod=Cartesian  TranslationLengthUnit=mm  TranslationStandardAxis=+Z  TranslationStandardOffset=0  TranslationCartesianOffset=[449.09427593857532 -79.972300000000033 18.776101630550443]  TranslationROffset=0  TranslationROffsetUnits=m  TranslationZOffset=0  TranslationZOffsetUnits=m  TranslationThetaOffset=0  TranslationThetaOffsetUnits=deg  RotationMethod=ArbitraryAxis  RotationAngleUnits=rad  RotationStandardAxis=+Z  RotationAngle=2.0943951023931953  RotationArbitraryAxis=[0.57735026918962551 0.57735026918962562 0.57735026918962606]  FollAlignAxisA=+X  BaseAlignAxisA=+Y  FollAlignAxisB=+Y  BaseAlignAxisB=+Z  BlockFunction=simmechanics.library.frames_transforms.rigid_transform
  Transform2 : sm_lib/Frames and Transforms/Rigid Transform  TranslationMethod=Cartesian  TranslationLengthUnit=mm  TranslationStandardAxis=+Z  TranslationStandardOffset=0  TranslationCartesianOffset=[55.8872 -79.97229999999999 18.7791]  TranslationROffset=0  TranslationROffsetUnits=m  TranslationZOffset=0  TranslationZOffsetUnits=m  TranslationThetaOffset=0  TranslationThetaOffsetUnits=deg  RotationMethod=ArbitraryAxis  RotationAngleUnits=rad  RotationStandardAxis=+Z  RotationAngle=1.6178481128137681  RotationArbitraryAxis=[0.21194708467810197 -0.21194708467810194 0.95402141830930975]  FollAlignAxisA=+X  BaseAlignAxisA=+Y  FollAlignAxisB=+Y  BaseAlignAxisB=+Z  BlockFunction=simmechanics.library.frames_transforms.rigid_transform
  Transform3 : sm_lib/Frames and Transforms/Rigid Transform  TranslationMethod=Cartesian  TranslationLengthUnit=mm  TranslationStandardAxis=+Z  TranslationStandardOffset=0  TranslationCartesianOffset=[111.887 -79.97229999999999 18.7791]  TranslationROffset=0  TranslationROffsetUnits=m  TranslationZOffset=0  TranslationZOffsetUnits=m  TranslationThetaOffset=0  TranslationThetaOffsetUnits=deg  RotationMethod=ArbitraryAxis  RotationAngleUnits=rad  RotationStandardAxis=+Z  RotationAngle=3.1415926535897931  RotationArbitraryAxis=[0 0.36955459314218925 0.92920901991291016]  FollAlignAxisA=+X  BaseAlignAxisA=+Y  FollAlignAxisB=+Y  BaseAlignAxisB=+Z  BlockFunction=simmechanics.library.frames_transforms.rigid_transform
  Transform4 : sm_lib/Frames and Transforms/Rigid Transform  TranslationMethod=Cartesian  TranslationLengthUnit=mm  TranslationStandardAxis=+Z  TranslationStandardOffset=0  TranslationCartesianOffset=[217.98699999999999 -6.5523399999999992 18.7791]  TranslationROffset=0  TranslationROffsetUnits=m  TranslationZOffset=0  TranslationZOffsetUnits=m  TranslationThetaOffset=0  TranslationThetaOffsetUnits=deg  RotationMethod=ArbitraryAxis  RotationAngleUnits=rad  RotationStandardAxis=+Z  RotationAngle=2.0943951023931953  RotationArbitraryAxis=[0.57735026918962584 0.57735026918962584 0.57735026918962584]  FollAlignAxisA=+X  BaseAlignAxisA=+Y  FollAlignAxisB=+Y  BaseAlignAxisB=+Z  BlockFunction=simmechanics.library.frames_transforms.rigid_transform
  Transform5 : sm_lib/Frames and Transforms/Rigid Transform  TranslationMethod=Cartesian  TranslationLengthUnit=mm  TranslationStandardAxis=+Z  TranslationStandardOffset=0  TranslationCartesianOffset=[16.944099999999999 -79.97229999999999 18.7791]  TranslationROffset=0  TranslationROffsetUnits=m  TranslationZOffset=0  TranslationZOffsetUnits=m  TranslationThetaOffset=0  TranslationThetaOffsetUnits=deg  RotationMethod=None  RotationAngleUnits=deg  RotationStandardAxis=+Z  RotationAngle=0  RotationArbitraryAxis=[0 0 1]  FollAlignAxisA=+X  BaseAlignAxisA=+Y  FollAlignAxisB=+Y  BaseAlignAxisB=+Z  BlockFunction=simmechanics.library.frames_transforms.rigid_transform
  x15060_Ecrou_24_Ecrou_Hm_M16_1_RIGID : Subsystem
  x15060_M_01073_Interface_ar_verin_AA_DEFAULT_1_RIGID : Subsystem
  x15060_NLM_Embout_a_rotule_M16_Pas_a_droite_27627_16_1_RIGID : Subsystem
  x15060_Verin_LA36_Course_100_mm_1_RIGID : Subsystem
  F1 : PMIOPort  Port=1  Side=Left
  F : PMIOPort  Port=2  Side=Left
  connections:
  Transform/LConn1 -- ReferenceFrame/RConn1 -- Transform1/LConn1 -- Transform2/LConn1 -- Transform3/LConn1 -- Transform4/LConn1 -- Transform5/LConn1
  Transform/RConn1 -- F/RConn1
  Transform1/RConn1 -- F1/RConn1
  Transform2/RConn1 -- x15060_Ecrou_24_Ecrou_Hm_M16_1_RIGID/LConn1
  Transform3/RConn1 -- x15060_M_01073_Interface_ar_verin_AA_DEFAULT_1_RIGID/LConn1
  Transform4/RConn1 -- x15060_Verin_LA36_Course_100_mm_1_RIGID/LConn1
  Transform5/RConn1 -- x15060_NLM_Embout_a_rotule_M16_Pas_a_droite_27627_16_1_RIGID/LConn1
